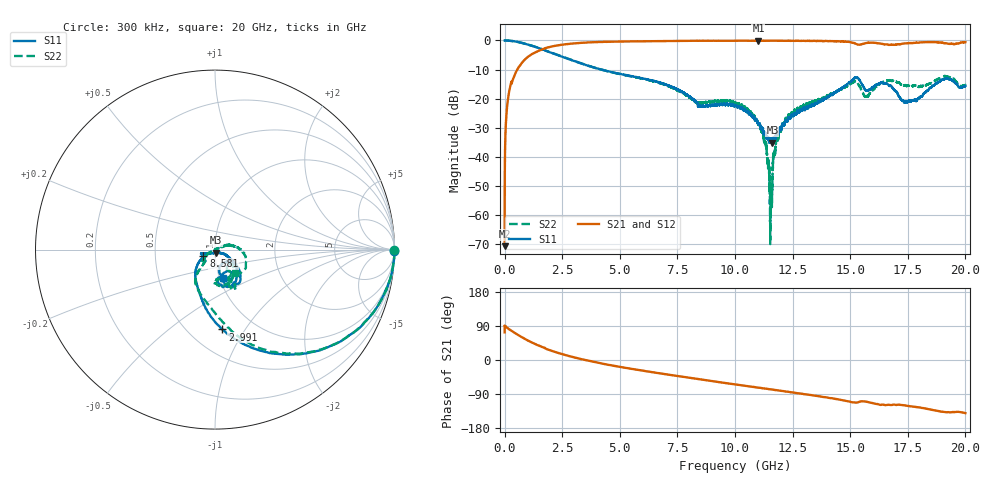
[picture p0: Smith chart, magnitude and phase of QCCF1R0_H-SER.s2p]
! Created Mon Feb  8 13:51:47 2021
# hz S ma R 50
! 2 Port Network Data from SP1.SP block
! freq  magS11  angS11  magS21  angS21  magS12  angS12  magS22  angS22
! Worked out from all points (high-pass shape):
!   20001 points, 300 kHz to 20 GHz, reference 50 ohm
!   highest |S21| = -0.08 dB at 11.02 GHz (marker M1); lowest = -70.7 dB at 300 kHz (marker M2)
!   |S21| within 3 dB of the highest: 1.633163 GHz to 1.633449 GHz (286.6 kHz wide, 0.0175 % of centre); 1.634 GHz to end of sweep
!   lowest |S11| = -35.2 dB at 11.62 GHz (marker M3), VSWR 1.04, Z = 50.4 - j1.71 ohm
!   |S11| at or under -10 dB: 4.177727 GHz to 4.178701 GHz (974 kHz wide, 0.0233 % of centre); 4.181974 GHz to 4.182805 GHz (830.1 kHz wide, 0.0198 % of centre); 4.184 GHz to end of sweep
!   |S22| runs from -70.0 to 0.0 dB; largest |S21 - S12| = 0.011
!   S11 on the Smith chart (normalised r, x): 300 kHz: open; 2.991 GHz: 0.72, -0.80; 8.581 GHz: 0.88, -0.06; 20 GHz: 1.04, -0.34
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300000  0.9982 -0.4  0.0002902 73.0  0.0002667 83.8  0.9986 -0.2
1.333e8  0.9954 -6.3  0.08961 84.0  0.08963 84.1  0.9956 -6.2
4.793e8  0.9576 -19.6  0.2789 70.1  0.2786 70.0  0.9584 -19.5
1.4063e9  0.7571 -50.2  0.6462 40.0  0.6464 40.0  0.7592 -49.2
2.9913e9  0.4467 -84.8  0.8875 7.5  0.8895 7.4  0.4508 -79.3
3.3343e9  0.4019 -90.1  0.9106 2.2  0.9104 2.2  0.404 -84.2
6.6673e9  0.1921 -124.6  0.975 -34.5  0.9759 -34.5  0.1882 -124.5
8.5813e9  0.07401 -151.4  0.988 -52.0  0.9889 -51.9  0.08576 -137.5
1.00003e10  0.07485 -162.8  0.9863 -64.4  0.9886 -64.4  0.08575 -141.2
1.10173e10  0.03675 -146.6  0.9912 -73.0  0.989 -73.0  0.0357 -151.1
1.12933e10  0.02478 -128.0  0.9892 -75.3  0.9888 -75.3  0.01771 -155.5
1.15223e10  0.019 -95.2  0.9907 -77.2  0.9883 -77.2  0.0009259 -146.7
1.16233e10  0.01739 -77.3  0.9867 -78.0  0.9875 -78.1  0.003991 18.8
1.17403e10  0.02063 -58.4  0.9886 -79.2  0.9897 -79.2  0.01224 26.5
1.20033e10  0.03004 -36.2  0.9884 -81.4  0.9883 -81.4  0.02887 22.5
1.33343e10  0.07609 -27.0  0.9815 -92.9  0.9821 -93.0  0.08541 15.5
1.52303e10  0.2282 -56.1  0.8807 -112.5  0.8794 -112.6  0.1966 -34.7
1.57003e10  0.1383 -67.2  0.9025 -110.0  0.9032 -110.0  0.1111 -47.4
1.66673e10  0.17 -71.4  0.8414 -118.1  0.8433 -118.5  0.2049 -74.7
1.74113e10  0.08788 -60.1  0.8925 -120.2  0.8933 -120.3  0.169 -86.9
1.90993e10  0.2167 -63.0  0.896 -137.6  0.9041 -137.7  0.2451 -62.7
2e10  0.1652 -73.7  0.9384 -140.2  0.933 -140.1  0.1721 -48.1
